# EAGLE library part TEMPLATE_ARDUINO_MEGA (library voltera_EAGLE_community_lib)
Use SHIELD for integrating into circuits. Use RAW for created the template boards.
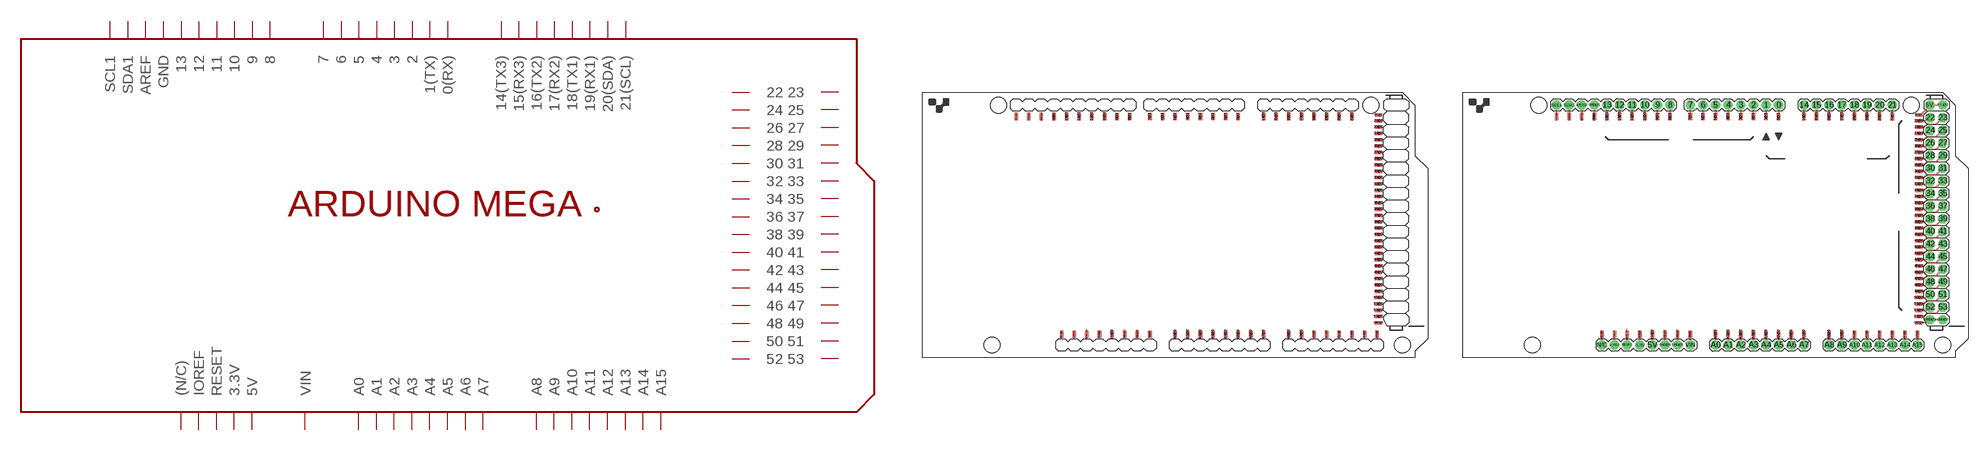
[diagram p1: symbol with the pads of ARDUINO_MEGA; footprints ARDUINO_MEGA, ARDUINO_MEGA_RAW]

Designator prefix P

## TEMPLATE_ARDUINO_MEGA_SHIELD  [ARDUINO_MEGA]
0@1  0(RX)
0@2  0(RX)
1@1  1(TX)
1@2  1(TX)
2@1  2
2@2  2
3@1  3
3@2  3
3V3@1  3.3V
3V3@2  3.3V
4@1  4
4@2  4
5@1  5
5@2  5
5V.@1  5V
5V.@3  5V
5V@1  5V
5V@2  5V
6@1  6
6@2  6
7@1  7
7@2  7
8@1  8
8@2  8
9@1  9
9@2  9
10@1  10
10@2  10
11@1  11
11@2  11
12@1  12
12@2  12
13@1  13
13@2  13
14@1  14(TX3)
14@2  14(TX3)
15@1  15(RX3)
15@2  15(RX3)
16@1  16(TX2)
16@2  16(TX2)
17@1  17(RX2)
17@2  17(RX2)
18@1  18(TX1)
18@2  18(TX1)
19@1  19(RX1)
19@2  19(RX1)
20@1  20(SDA)
20@2  20(SDA)
21@1  21(SCL)
21@2  21(SCL)
22@1  22
22@2  22
23@1  23
23@2  23
24@1  24
24@2  24
25@1  25
25@2  25
26@1  26
26@2  26
27@1  27
27@2  27
28@1  28
28@2  28
29@1  29
29@2  29
30@1  30
30@2  30
31@1  31
31@2  31
32@1  32
32@2  32
33@1  33
33@2  33
34@1  34
34@2  34
35@1  35
35@2  35
36@1  36
36@2  36
37@1  37
37@2  37
38@1  38
38@2  38
39@1  39
39@2  39
40@1  40
40@2  40
41@1  41
41@2  41
42@1  42
42@2  42
43@1  43
43@2  43
44@1  44
44@2  44
45@1  45
45@2  45
46@1  46
46@2  46
47@1  47
47@2  47
48@1  48
48@2  48
49@1  49
49@2  49
50@1  50
50@2  50
51@1  51
51@2  51
52@1  52
52@2  52
53@1  53
53@2  53
A0@1  A0
A0@2  A0
A1@1  A1
A1@2  A1
A2@1  A2
A2@2  A2
A3@1  A3
A3@2  A3
A4@1  A4
A4@2  A4
A5@1  A5
A5@2  A5
A6@1  A6
A6@2  A6
A7@1  A7
A7@2  A7
A8@1  A8
A8@2  A8
A9@1  A9
A9@2  A9
A10@1  A10
A10@2  A10
A11@1  A11
A11@2  A11
A12@1  A12
A12@2  A12
A13@1  A13
A13@2  A13
A14@1  A14
A14@2  A14
A15@1  A15
A15@2  A15
AREF@1  AREF
AREF@2  AREF
GND  GND
GND1  GND
GND@4  GND
GND@7  GND
GND@8  GND
GND@9  GND
GND@10  GND
GND@11  GND
I/OREF@1  IOREF
I/OREF@2  IOREF
N/C@1  (N/C)
N/C@2  (N/C)
RESET@1  RESET
RESET@2  RESET
SCL1@1  SCL1
SCL1@2  SCL1
SDA1@1  SDA1
SDA1@2  SDA1
VIN@1  VIN
VIN@2  VIN

## TEMPLATE_ARDUINO_MEGA_RAW  [ARDUINO_MEGA_RAW]
0  0(RX)
0@1  0(RX)
0@2  0(RX)
1  1(TX)
1@1  1(TX)
1@2  1(TX)
2  2
2@1  2
2@2  2
3  3
3.3V  3.3V
3@1  3
3@2  3
3V3@1  3.3V
3V3@2  3.3V
4  4
4@1  4
4@2  4
5  5
5@1  5
5@2  5
5V  5V
5V.  5V
5V.@1  5V
5V.@2  5V
5V.@3  5V
5V@1  5V
5V@2  5V
6  6
6@1  6
6@2  6
7  7
7@1  7
7@2  7
8  8
8@1  8
8@2  8
9  9
9@1  9
9@2  9
10  10
10@1  10
10@2  10
11  11
11@1  11
11@2  11
12  12
12@1  12
12@2  12
13  13
13@1  13
13@2  13
14  14(TX3)
14@1  14(TX3)
14@2  14(TX3)
15  15(RX3)
15@1  15(RX3)
15@2  15(RX3)
16  16(TX2)
16@1  16(TX2)
16@2  16(TX2)
17  17(RX2)
17@1  17(RX2)
17@2  17(RX2)
18  18(TX1)
18@1  18(TX1)
18@2  18(TX1)
19  19(RX1)
19@1  19(RX1)
19@2  19(RX1)
20  20(SDA)
20@1  20(SDA)
20@2  20(SDA)
21  21(SCL)
21@1  21(SCL)
21@2  21(SCL)
22  22
22@1  22
22@2  22
23  23
23@1  23
23@2  23
24  24
24@1  24
24@2  24
25  25
25@1  25
25@2  25
26  26
26@1  26
26@2  26
27  27
27@1  27
27@2  27
28  28
28@1  28
28@2  28
29  29
29@1  29
29@2  29
30  30
30@1  30
30@2  30
31  31
31@1  31
31@2  31
32  32
32@1  32
32@2  32
33  33
33@1  33
33@2  33
34  34
34@1  34
34@2  34
35  35
35@1  35
35@2  35
36  36
36@1  36
36@2  36
37  37
37@1  37
37@2  37
38  38
38@1  38
38@2  38
39  39
39@1  39
39@2  39
40  40
40@1  40
40@2  40
41  41
41@1  41
41@2  41
42  42
42@1  42
42@2  42
43  43
43@1  43
43@2  43
44  44
44@1  44
44@2  44
45  45
45@1  45
45@2  45
46  46
46@1  46
46@2  46
47  47
47@1  47
47@2  47
48  48
48@1  48
48@2  48
49  49
49@1  49
49@2  49
50  50
50@1  50
50@2  50
51  51
51@1  51
51@2  51
52  52
52@1  52
52@2  52
53  53
53@1  53
53@2  53
A0  A0
A0@1  A0
A0@2  A0
A1  A1
A1@1  A1
A1@2  A1
A2  A2
A2@1  A2
A2@2  A2
A3  A3
A3@1  A3
A3@2  A3
A4  A4
A4@1  A4
A4@2  A4
A5  A5
A5@1  A5
A5@2  A5
A6  A6
A6@1  A6
A6@2  A6
A7  A7
A7@1  A7
A7@2  A7
A8  A8
A8@1  A8
A8@2  A8
A9  A9
A9@1  A9
A9@2  A9
A10  A10
A10@1  A10
A10@2  A10
A11  A11
A11@1  A11
A11@2  A11
A12  A12
A12@1  A12
A12@2  A12
A13  A13
A13@1  A13
A13@2  A13
A14  A14
A14@1  A14
A14@2  A14
A15  A15
A15@1  A15
A15@2  A15
AREF  AREF
AREF@1  AREF
AREF@2  AREF
GND  GND
GND1  GND
GND@1  GND
GND@2  GND
GND@3  GND
GND@4  GND
GND@5  GND
GND@6  GND
GND@7  GND
GND@8  GND
GND@9  GND
GND@10  GND
GND@11  GND
I/OREF  IOREF
I/OREF@1  IOREF
I/OREF@2  IOREF
N/C  (N/C)
N/C@1  (N/C)
N/C@2  (N/C)
RESET  RESET
RESET@1  RESET
RESET@2  RESET
SCL1  SCL1
SCL1@1  SCL1
SCL1@2  SCL1
SDA1  SDA1
SDA1@1  SDA1
SDA1@2  SDA1
VIN  VIN
VIN@1  VIN
VIN@2  VIN

## Footprint ARDUINO_MEGA (pad centres in mm)
Footprint for representing an Arduino Mega board in an EAGLE schematic. Created by Dave Young for Element14. More EAGLE documentation at: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
smd 0.711 x 1.422 bottom: 0@1 63.5,48.5; 1@1 60.96,48.5; 2@1 58.42,48.5; 3@1 55.88,48.5; 3V3@1 35.56,4.713; 4@1 53.34,48.5; 5@1 50.8,48.5; 5V@1 38.1,4.713; 6@1 48.26,48.5; 7@1 45.72,48.5; 8@1 41.656,48.5; 9@1 39.116,48.5; 10@1 36.576,48.5; 11@1 34.036,48.5; 12@1 31.496,48.5; 13@1 28.956,48.5; 14@1 68.58,48.5; 15@1 71.12,48.5; 16@1 73.66,48.5; 17@1 76.2,48.5; 18@1 78.74,48.5; 19@1 81.28,48.5; 20@1 83.82,48.5; 21@1 86.36,48.5; A0@1 50.8,4.713; A1@1 53.34,4.713; A2@1 55.88,4.713; A3@1 58.42,4.713; A4@1 60.96,4.713; A5@1 63.5,4.713; A6@1 66.04,4.713; A7@1 68.58,4.713; A8@1 73.66,4.713; A9@1 76.2,4.713; A10@1 78.74,4.713; A11@1 81.28,4.713; A12@1 83.82,4.713; A13@1 86.36,4.713; A14@1 88.9,4.713; A15@1 91.44,4.713; AREF@1 23.876,48.5; GND 26.416,48.5; GND@7 40.64,4.713; GND@8 43.18,4.713; I/OREF@1 30.48,4.713; N/C@1 27.94,4.713; RESET@1 33.02,4.713; SCL1@1 18.796,48.5; SDA1@1 21.336,48.5; VIN@1 45.72,4.713
smd 0.711 x 1.422: 0@2 63.5,48.5; 1@2 60.96,48.5; 2@2 58.42,48.5; 3@2 55.88,48.5; 3V3@2 35.56,4.713; 4@2 53.34,48.5; 5@2 50.8,48.5; 5V@2 38.1,4.713; 6@2 48.26,48.5; 7@2 45.72,48.5; 8@2 41.656,48.5; 9@2 39.116,48.5; 10@2 36.576,48.5; 11@2 34.036,48.5; 12@2 31.496,48.5; 13@2 28.956,48.5; 14@2 68.58,48.5; 15@2 71.12,48.5; 16@2 73.66,48.5; 17@2 76.2,48.5; 18@2 78.74,48.5; 19@2 81.28,48.5; 20@2 83.82,48.5; 21@2 86.36,48.5; A0@2 50.8,4.713; A1@2 53.34,4.713; A2@2 55.88,4.713; A3@2 58.42,4.713; A4@2 60.96,4.713; A5@2 63.5,4.713; A6@2 66.04,4.713; A7@2 68.58,4.713; A8@2 73.66,4.713; A9@2 76.2,4.713; A10@2 78.74,4.713; A11@2 81.28,4.713; A12@2 83.82,4.713; A13@2 86.36,4.713; A14@2 88.9,4.713; A15@2 91.44,4.713; AREF@2 23.876,48.5; GND1 26.416,48.5; GND@10 40.64,4.713; GND@11 43.18,4.713; I/OREF@2 30.48,4.713; N/C@2 27.94,4.713; RESET@2 33.02,4.713; SCL1@2 18.796,48.5; SDA1@2 21.336,48.5; VIN@2 45.72,4.713
smd 1.422 x 0.711 bottom: 5V.@1 91.669,48.768; 22@1 91.669,47.625; 23@1 91.669,46.355; 24@1 91.669,45.085; 25@1 91.669,43.815; 26@1 91.669,42.545; 27@1 91.669,41.275; 28@1 91.669,40.005; 29@1 91.669,38.735; 30@1 91.669,37.465; 31@1 91.669,36.195; 32@1 91.669,34.925; 33@1 91.669,33.655; 34@1 91.669,32.385; 35@1 91.669,31.115; 36@1 91.669,29.845; 37@1 91.669,28.575; 38@1 91.669,27.305; 39@1 91.669,26.035; 40@1 91.669,24.765; 41@1 91.669,23.495; 42@1 91.669,22.225; 43@1 91.669,20.955; 44@1 91.669,19.685; 45@1 91.669,18.415; 46@1 91.669,17.145; 47@1 91.669,15.875; 48@1 91.669,14.605; 49@1 91.669,13.335; 50@1 91.669,12.065; 51@1 91.669,10.795; 52@1 91.669,9.525; 53@1 91.669,8.255; GND@4 91.669,6.985
smd 1.422 x 0.711: 5V.@3 91.669,48.768; 22@2 91.669,47.625; 23@2 91.669,46.355; 24@2 91.669,45.085; 25@2 91.669,43.815; 26@2 91.669,42.545; 27@2 91.669,41.275; 28@2 91.669,40.005; 29@2 91.669,38.735; 30@2 91.669,37.465; 31@2 91.669,36.195; 32@2 91.669,34.925; 33@2 91.669,33.655; 34@2 91.669,32.385; 35@2 91.669,31.115; 36@2 91.669,29.845; 37@2 91.669,28.575; 38@2 91.669,27.305; 39@2 91.669,26.035; 40@2 91.669,24.765; 41@2 91.669,23.495; 42@2 91.669,22.225; 43@2 91.669,20.955; 44@2 91.669,19.685; 45@2 91.669,18.415; 46@2 91.669,17.145; 47@2 91.669,15.875; 48@2 91.669,14.605; 49@2 91.669,13.335; 50@2 91.669,12.065; 51@2 91.669,10.795; 52@2 91.669,9.525; 53@2 91.669,8.255; GND@9 91.669,6.985
hole 3.2 at 15.24,50.8
hole 3.2 at 13.97,2.54
hole 3.2 at 90.17,50.8
hole 3.2 at 96.52,2.54

## Footprint ARDUINO_MEGA_RAW (pad centres in mm)
Footprint for representing an Arduino Mega board in an EAGLE schematic. Created by Dave Young for Element14. More EAGLE documentation at: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
drill 1.016 pad 1.88: 0 63.5,50.8; 1 60.96,50.8; 2 58.42,50.8; 3 55.88,50.8; 3.3V 35.56,2.54; 4 53.34,50.8; 5 50.8,50.8; 5V 38.1,2.54; 5V. 93.98,50.8; 5V.@2 96.52,50.8; 6 48.26,50.8; 7 45.72,50.8; 8 41.656,50.8; 9 39.116,50.8; 10 36.576,50.8; 11 34.036,50.8; 12 31.496,50.8; 13 28.956,50.8; 14 68.58,50.8; 15 71.12,50.8; 16 73.66,50.8; 17 76.2,50.8; 18 78.74,50.8; 19 81.28,50.8; 20 83.82,50.8; 21 86.36,50.8; A0 50.8,2.54; A1 53.34,2.54; A2 55.88,2.54; A3 58.42,2.54; A4 60.96,2.54; A5 63.5,2.54; A6 66.04,2.54; A7 68.58,2.54; A8 73.66,2.54; A9 76.2,2.54; A10 78.74,2.54; A11 81.28,2.54; A12 83.82,2.54; A13 86.36,2.54; A14 88.9,2.54; A15 91.44,2.54; AREF 23.876,50.8; GND@1 26.416,50.8; GND@2 96.52,7.62; GND@3 93.98,7.62; GND@5 43.18,2.54; GND@6 40.64,2.54; I/OREF 30.48,2.54; N/C 27.94,2.54; RESET 33.02,2.54; SCL1 18.796,50.8; SDA1 21.336,50.8; VIN 45.72,2.54
smd 0.711 x 1.422 bottom: 0@1 63.5,48.5; 1@1 60.96,48.5; 2@1 58.42,48.5; 3@1 55.88,48.5; 3V3@1 35.56,4.713; 4@1 53.34,48.5; 5@1 50.8,48.5; 5V@1 38.1,4.713; 6@1 48.26,48.5; 7@1 45.72,48.5; 8@1 41.656,48.5; 9@1 39.116,48.5; 10@1 36.576,48.5; 11@1 34.036,48.5; 12@1 31.496,48.5; 13@1 28.956,48.5; 14@1 68.58,48.5; 15@1 71.12,48.5; 16@1 73.66,48.5; 17@1 76.2,48.5; 18@1 78.74,48.5; 19@1 81.28,48.5; 20@1 83.82,48.5; 21@1 86.36,48.5; A0@1 50.8,4.713; A1@1 53.34,4.713; A2@1 55.88,4.713; A3@1 58.42,4.713; A4@1 60.96,4.713; A5@1 63.5,4.713; A6@1 66.04,4.713; A7@1 68.58,4.713; A8@1 73.66,4.713; A9@1 76.2,4.713; A10@1 78.74,4.713; A11@1 81.28,4.713; A12@1 83.82,4.713; A13@1 86.36,4.713; A14@1 88.9,4.713; A15@1 91.44,4.713; AREF@1 23.876,48.5; GND 26.416,48.5; GND@7 40.64,4.713; GND@8 43.18,4.713; I/OREF@1 30.48,4.713; N/C@1 27.94,4.713; RESET@1 33.02,4.713; SCL1@1 18.796,48.5; SDA1@1 21.336,48.5; VIN@1 45.72,4.713
smd 0.711 x 1.422: 0@2 63.5,48.5; 1@2 60.96,48.5; 2@2 58.42,48.5; 3@2 55.88,48.5; 3V3@2 35.56,4.713; 4@2 53.34,48.5; 5@2 50.8,48.5; 5V@2 38.1,4.713; 6@2 48.26,48.5; 7@2 45.72,48.5; 8@2 41.656,48.5; 9@2 39.116,48.5; 10@2 36.576,48.5; 11@2 34.036,48.5; 12@2 31.496,48.5; 13@2 28.956,48.5; 14@2 68.58,48.5; 15@2 71.12,48.5; 16@2 73.66,48.5; 17@2 76.2,48.5; 18@2 78.74,48.5; 19@2 81.28,48.5; 20@2 83.82,48.5; 21@2 86.36,48.5; A0@2 50.8,4.713; A1@2 53.34,4.713; A2@2 55.88,4.713; A3@2 58.42,4.713; A4@2 60.96,4.713; A5@2 63.5,4.713; A6@2 66.04,4.713; A7@2 68.58,4.713; A8@2 73.66,4.713; A9@2 76.2,4.713; A10@2 78.74,4.713; A11@2 81.28,4.713; A12@2 83.82,4.713; A13@2 86.36,4.713; A14@2 88.9,4.713; A15@2 91.44,4.713; AREF@2 23.876,48.5; GND1 26.416,48.5; GND@10 40.64,4.713; GND@11 43.18,4.713; I/OREF@2 30.48,4.713; N/C@2 27.94,4.713; RESET@2 33.02,4.713; SCL1@2 18.796,48.5; SDA1@2 21.336,48.5; VIN@2 45.72,4.713
smd 1.422 x 0.711 bottom: 5V.@1 91.669,48.768; 22@1 91.669,47.625; 23@1 91.669,46.355; 24@1 91.669,45.085; 25@1 91.669,43.815; 26@1 91.669,42.545; 27@1 91.669,41.275; 28@1 91.669,40.005; 29@1 91.669,38.735; 30@1 91.669,37.465; 31@1 91.669,36.195; 32@1 91.669,34.925; 33@1 91.669,33.655; 34@1 91.669,32.385; 35@1 91.669,31.115; 36@1 91.669,29.845; 37@1 91.669,28.575; 38@1 91.669,27.305; 39@1 91.669,26.035; 40@1 91.669,24.765; 41@1 91.669,23.495; 42@1 91.669,22.225; 43@1 91.669,20.955; 44@1 91.669,19.685; 45@1 91.669,18.415; 46@1 91.669,17.145; 47@1 91.669,15.875; 48@1 91.669,14.605; 49@1 91.669,13.335; 50@1 91.669,12.065; 51@1 91.669,10.795; 52@1 91.669,9.525; 53@1 91.669,8.255; GND@4 91.669,6.985
smd 1.422 x 0.711: 5V.@3 91.669,48.768; 22@2 91.669,47.625; 23@2 91.669,46.355; 24@2 91.669,45.085; 25@2 91.669,43.815; 26@2 91.669,42.545; 27@2 91.669,41.275; 28@2 91.669,40.005; 29@2 91.669,38.735; 30@2 91.669,37.465; 31@2 91.669,36.195; 32@2 91.669,34.925; 33@2 91.669,33.655; 34@2 91.669,32.385; 35@2 91.669,31.115; 36@2 91.669,29.845; 37@2 91.669,28.575; 38@2 91.669,27.305; 39@2 91.669,26.035; 40@2 91.669,24.765; 41@2 91.669,23.495; 42@2 91.669,22.225; 43@2 91.669,20.955; 44@2 91.669,19.685; 45@2 91.669,18.415; 46@2 91.669,17.145; 47@2 91.669,15.875; 48@2 91.669,14.605; 49@2 91.669,13.335; 50@2 91.669,12.065; 51@2 91.669,10.795; 52@2 91.669,9.525; 53@2 91.669,8.255; GND@9 91.669,6.985
drill 1.016 pad 1.88 octagon: 22 93.98,48.26; 23 96.52,48.26; 24 93.98,45.72; 25 96.52,45.72; 26 93.98,43.18; 27 96.52,43.18; 28 93.98,40.64; 29 96.52,40.64; 30 93.98,38.1; 31 96.52,38.1; 32 93.98,35.56; 33 96.52,35.56; 34 93.98,33.02; 35 96.52,33.02; 36 93.98,30.48; 37 96.52,30.48; 38 93.98,27.94; 39 96.52,27.94; 40 93.98,25.4; 41 96.52,25.4; 42 93.98,22.86; 43 96.52,22.86; 44 93.98,20.32; 45 96.52,20.32; 46 93.98,17.78; 47 96.52,17.78; 48 93.98,15.24; 49 96.52,15.24; 50 93.98,12.7; 51 96.52,12.7; 52 93.98,10.16; 53 96.52,10.16
hole 3.2 at 15.24,50.8
hole 3.2 at 13.97,2.54
hole 3.2 at 90.17,50.8
hole 3.2 at 96.52,2.54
